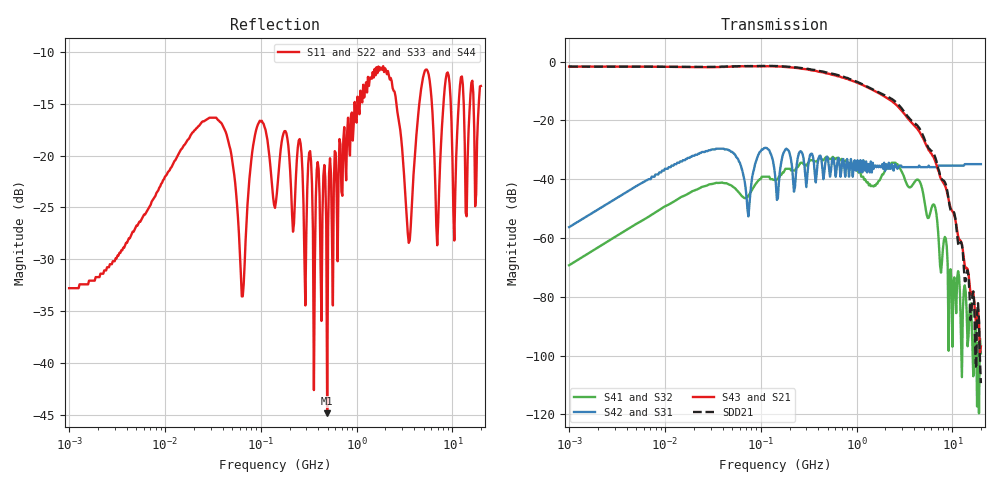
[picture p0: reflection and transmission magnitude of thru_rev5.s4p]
# MHZ S MA R 50
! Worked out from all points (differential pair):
!   435 points, 1 MHz to 19.82 GHz, reference 50 ohm
!   strongest paths, dB at 1 MHz, 11.73 MHz, 140.8 MHz, 1.689 GHz, 19.82 GHz:
!     S43: -1.7, -1.8, -1.6, -10.7, -96.9
!     S21: -1.7, -1.8, -1.6, -10.7, -96.9
!     S42: -56.3, -35.4, -38.4, -35.9, -34.9
!     S31: -56.3, -35.4, -38.4, -35.9, -34.9
!     S41: -69.3, -48.1, -40.3, -40.7, -99.3
!     S32: -69.3, -48.1, -40.3, -40.7, -99.3
!   taken as a pair (ports 3,1 in; 4,2 out), SDD21 dB: -1.7, -1.8, -1.5, -10.4, -109.4
!   lowest |S11| = -44.8 dB at 493.3 MHz (marker M1), VSWR 1.01, Z = 49.7 - j0.512 ohm
!   |S11| at or under -10 dB: start of sweep to end of sweep
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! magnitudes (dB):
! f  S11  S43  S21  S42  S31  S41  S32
! 1 MHz  -32.8  -1.7  -1.7  -56.3  -56.3  -69.3  -69.3
! 29.87 MHz  -16.4  -1.9  -1.9  -30.2  -30.2  -41.7  -41.7
! 74.35 MHz  -23.5  -1.6  -1.6  -52.7  -52.7  -45.7  -45.7
! 493.3 MHz  -44.8  -4.0  -4.0  -32.4  -32.4  -32.4  -32.4
! 4.401 GHz  -16.0  -23.3  -23.3  -35.9  -35.9  -40.2  -40.2
! 9.554 GHz  -14.5  -49.7  -49.7  -35.4  -35.4  -70.6  -70.6
! 19.82 GHz  -13.3  -96.9  -96.9  -34.9  -34.9  -99.3  -99.3
